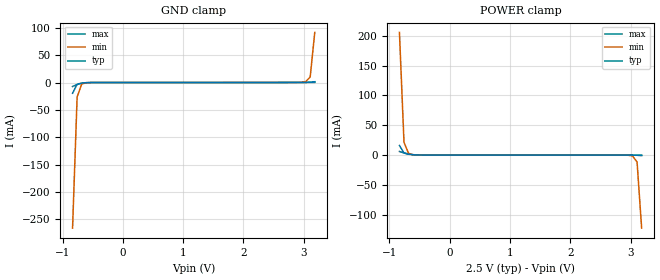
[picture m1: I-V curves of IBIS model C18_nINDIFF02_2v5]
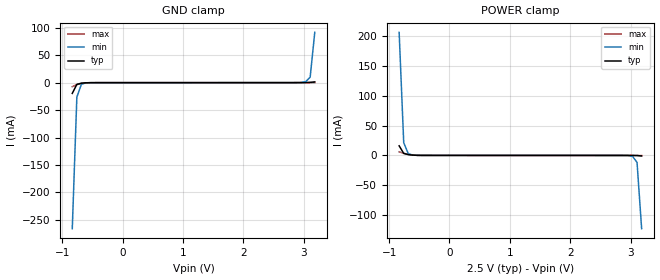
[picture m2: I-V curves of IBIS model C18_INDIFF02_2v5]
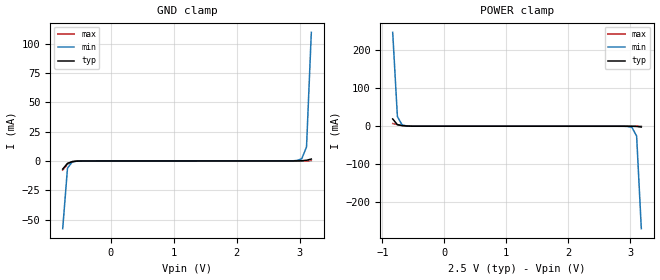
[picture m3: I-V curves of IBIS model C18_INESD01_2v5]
|   This file is an IBIS representation of the   |
|   Integrated Device Technology, Inc.   |
|   8L30210I   |
|   CRYSTAL OR DIFFERENTIAL-TO-LVCMOS LVTTL CLOCK BUFFER   |
[IBIS Ver]   4.1
[File name]   8l30210i.ibs
[File Rev]   1.0
[Date]   04 Dec 2019
[Source]   Originated at Integrated Device Technology, Inc.
[Disclaimer]
IDT hereby grants the user of this IBIS model a non-exclusive,
nontransferable license to use this IBIS model under the following terms.
Before using this IBIS model, the user should read this license.
If the user does not accept these terms,  the IBIS model should be
returned to IDT within 30 days.
   The user is granted this license only to use the IBIS model and
is not granted rights to sell, load, rent, lease or license the IBIS
model in whole or in part, or in modified form to anyone other than
user. User may modify the IBIS model to suit its specific
applications but rights to derivative works and such modifications
shall belong to IDT.
   This IBIS model is provided on an "AS IS" basis and IDT makes
absolutely no warranty with respect to the information contained
herein. IDT DISCLAIMS AND CUSTOMER WAIVES ALL WARRANTIES, EXPRESS
OR IMPLIED, INCLUDING WARRANTIES OF MERCHANTABILITY OR FITNESS FOR
A PARTICULAR PURPOSE. The entire risk as to quality and performance
is with the Customer. ACCORDINGLY, IN NO EVENT SHALL THE COMPANY BE
LIABLE FOR ANY DAMAGES, WHETHER IN CONTRACT OR TORT,INCLUDING ANY
LOST PROFITS OR OTHER INCIDENTAL, CONSEQUENTIAL, EXEMPLARY, OR
PUNITIVE DAMAGES ARISING OUT OF THE USE OR APPLICATION OF THE IBIS
model provided in this package. Further, IDT reserves the right to
make changes without notice to any product herein to improve
reliability, function, or design. IDT does not convey any license
under patent rights or any other intellectual property rights,
including those of third parties.
   IDT is not obligated to provide maintenance or support
for the licensed IBIS model.
[Copyright] Copyright 2019 by Integrated Device Technology, Inc.
[Component]   8L30210NLGI
[Manufacturer] Integrated Device Technology, Inc.
[Package]
|QFN 32
|lead + wire   typ   min   max
R_pkg   72.4655m   58.886m   86.045m
L_pkg   1.47175nH   1.11650nH   1.77850nH
C_pkg   0.07747pF   0.07444pF   0.08050pF
[Pin] signal_name   model_name   R_pin   L_pin   C_pin
1   Q0   c18_OCMOS50OHM09   86.045m   1.77850nH   0.08050pF
2   VDDO   POWER   76.996m   1.55783nH   0.07848pF
3   Q1   c18_OCMOS50OHM09   67.941m   1.33717nH   0.07646pF
4   GND0   GND   58.886m   1.11650nH   0.07444pF
5   Q2   c18_OCMOS50OHM09   58.886m   1.11650nH   0.07444pF
6   VDDO   POWER   67.941m   1.33717nH   0.07646pF
7   Q3   c18_OCMOS50OHM09   76.996m   1.55783nH   0.07848pF
8   Q4   c18_OCMOS50OHM09   86.045m   1.77850nH   0.08050pF
9   GND0   GND   86.045m   1.77850nH   0.08050pF
10   VDD   POWER   76.996m   1.55783nH   0.07848pF
11   XTAL_IN   NC   67.941m   1.33717nH   0.07646pF
12   XTAL_OUT   NC   58.886m   1.11650nH   0.07444pF
13   CLK0   C18_INDIFF02   58.886m   1.11650nH   0.07444pF
14   nCLK0   C18_nINDIFF02   67.941m   1.33717nH   0.07646pF
15   GND   GND   76.996m   1.55783nH   0.07848pF
16   GND0   GND   86.045m   1.77850nH   0.08050pF
17   Q5   c18_OCMOS50OHM09   86.045m   1.77850nH   0.08050pF
18   Q6   c18_OCMOS50OHM09   76.996m   1.55783nH   0.07848pF
19   VDD0   POWER   67.941m   1.33717nH   0.07646pF
20   Q7   c18_OCMOS50OHM09   58.886m   1.11650nH   0.07444pF
21   GND0   GND   58.886m   1.11650nH   0.07444pF
22   Q8   c18_OCMOS50OHM09   67.941m   1.33717nH   0.07646pF
23   VDDO   POWER   76.996m   1.55783nH   0.07848pF
24   Q9   c18_OCMOS50OHM09   86.045m   1.77850nH   0.08050pF
25   GND0   GND   86.045m   1.77850nH   0.08050pF
26   GND   GND   76.996m   1.55783nH   0.07848pF
27   nCLK1   C18_nINDIFF02   67.941m   1.33717nH   0.07646pF
28   CLK1   C18_INDIFF02   58.886m   1.11650nH   0.07444pF
29   SEL1   C18_INESD01   58.886m   1.11650nH   0.07444pF
30   SEL0   C18_INESD01   67.941m   1.33717nH   0.07646pF
31   OE   C18_INESD01   76.996m   1.55783nH   0.07848pF
32   GND0   GND   86.045m   1.77850nH   0.08050pF
[Diff Pin]  inv_pin  vdiff tdelay_typ tdelay_min  tdelay_max
13   14   0.15   NA   NA   NA
28   27   0.15   NA   NA   NA
[Model Selector] c18_OCMOS50OHM09
c18_OCMOS50OHM09_1v5  Buffer selection for 1v5
c18_OCMOS50OHM09_1v8  Buffer selection for 1v8
c18_OCMOS50OHM09_2v5  Buffer selection for 2v5
c18_OCMOS50OHM09_3v3  Buffer selection for 3v3
[Model Selector] C18_nINDIFF02
C18_nINDIFF02_2v5  Buffer selection for 2v5
C18_nINDIFF02_3v3  Buffer selection for 3v3
[Model Selector] C18_INDIFF02
C18_INDIFF02_2v5  Buffer selection for 2v5
C18_INDIFF02_3v3  Buffer selection for 3v3
[Model Selector] C18_INESD01
C18_INESD01_2v5  Buffer selection for 2v5
C18_INESD01_3v3  Buffer selection for 3v3
| Models and submodels in the file (10): C18_nINDIFF02_2v5 (Input), C18_INDIFF02_2v5 (Input), C18_INESD01_2v5 (Input), c18_OCMOS50OHM09_1v5 (Output), c18_OCMOS50OHM09_1v8 (Output), c18_OCMOS50OHM09_2v5 (Output), c18_OCMOS50OHM09_3v3 (Output), C18_nINDIFF02_3v3 (Input), C18_INDIFF02_3v3 (Input), C18_INESD01_3v3 (Input)
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[Model] C18_nINDIFF02_2v5
Model_type   Input
Polarity   Non-Inverting
Vinl = 0.7V
Vinh = 1.7V
|   typ   min   max
C_comp   2pF   1.5pF   2.5pF
|   typ   min   max
[Voltage range]   2.5V   2.375V   2.625V
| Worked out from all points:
|   GND clamp passes 1 mA (typ) near -0.68 V on its own axis
|   POWER clamp passes 1 mA (typ) near -0.65 V on its own axis
[GND_clamp]
|Voltage   I (typ)   I (min)   I (max)
|Note, modeling breaks down at 250mA and above.  This is well beyond the functional   |
|operating range of the device.  Should this scenario occur, catastrophic failure and   |
|possible damage to the device and/or board is of higher concern than the I-V curve   |
|behavior.  The IBIS checker will flag currents in excess of 10A with warnings.  Lines   |
|with currents in excess of 0.35 A have been commented out.  The points still remain|
|available to the user if the user desires to use them.   |
|-2.50000e+00   -1.17752e+01   -1.02957e+01   -1.42772e+01
|-2.42424e+00   -1.12274e+01   -9.83984e+00   -1.35771e+01
|-2.34848e+00   -1.06796e+01   -9.38392e+00   -1.28769e+01
|-2.27273e+00   -1.01318e+01   -8.92797e+00   -1.21767e+01
|-2.19697e+00   -9.58387e+00   -8.47198e+00   -1.14763e+01
|-2.12121e+00   -9.03588e+00   -8.01595e+00   -1.07758e+01
|-2.04545e+00   -8.48784e+00   -7.55989e+00   -1.00752e+01
|-1.96970e+00   -7.93974e+00   -7.10380e+00   -9.37454e+00
|-1.89394e+00   -7.39159e+00   -6.64768e+00   -8.67378e+00
|-1.81818e+00   -6.84339e+00   -6.19154e+00   -7.97293e+00
|-1.74242e+00   -6.29514e+00   -5.73539e+00   -7.27199e+00
|-1.66667e+00   -5.74687e+00   -5.27924e+00   -6.57098e+00
|-1.59091e+00   -5.19857e+00   -4.82308e+00   -5.86989e+00
|-1.51515e+00   -4.65027e+00   -4.36695e+00   -5.16875e+00
|-1.43939e+00   -4.10197e+00   -3.91083e+00   -4.46756e+00
|-1.36364e+00   -3.55369e+00   -3.45477e+00   -3.76634e+00
|-1.28788e+00   -3.00546e+00   -2.99876e+00   -3.06512e+00
|-1.21212e+00   -2.45731e+00   -2.54285e+00   -2.36393e+00
|-1.13636e+00   -1.90928e+00   -2.08704e+00   -1.66282e+00
|-1.06061e+00   -1.36142e+00   -1.63139e+00   -9.61838e-01
|-9.84848e-01   -8.13796e-01   -1.17595e+00   -2.61081e-01
|-9.09091e-01   -2.66503e-01   -7.20781e-01   -1.77649e-02
-833.3mV  -19.6mA    -266mA     -7.357mA
-757.6mV  -3.22mA    -26.35mA   -3.621mA
-681.8mV  -988.6uA   -2.843mA   -1.31mA
-530.3mV  -114.3uA   -121.3uA   -118.4uA
2.803V    62.2uA     69.71uA    63.29uA
3.03V     168.3uA    1.59mA     74.62uA
3.106V    527.5uA    10.07mA    99.45uA
3.182V    1.407mA    91.57mA    275.1uA
| 3.25758e+00   3.38287e-03   7.21084e-01   9.53838e-04
| 3.33333e+00   1.60717e-02   1.60186e+00   2.32699e-03
| 3.40909e+00   2.04604e-01   2.48284e+00   4.31441e-03
| 3.48485e+00   1.20201e+00   3.36401e+00   7.22826e-03
| 3.56061e+00   2.26050e+00   4.24535e+00   2.70580e-02
| 3.63636e+00   3.31920e+00   5.12684e+00   5.94903e-01
| 3.71212e+00   4.37810e+00   6.00848e+00   1.94867e+00
| 3.78788e+00   5.43717e+00   6.89026e+00   3.30270e+00
| 3.86364e+00   6.49642e+00   7.77218e+00   4.65695e+00
| 3.93939e+00   7.55581e+00   8.65422e+00   6.01139e+00
| 4.01515e+00   8.61535e+00   9.53640e+00   7.36602e+00
| 4.09091e+00   9.67503e+00   1.04187e+01   8.72081e+00
| 4.16667e+00   1.07348e+01   1.13011e+01   1.00758e+01
| 4.24242e+00   1.17948e+01   1.21837e+01   1.14308e+01
| 4.31818e+00   1.28549e+01   1.30664e+01   1.27860e+01
| 4.39394e+00   1.39151e+01   1.39493e+01   1.41414e+01
| 4.46970e+00   1.49754e+01   1.48323e+01   1.54969e+01
| 4.54545e+00   1.60359e+01   1.57155e+01   1.68525e+01
| 4.62121e+00   1.70966e+01   1.65988e+01   1.82082e+01
| 4.69697e+00   1.81574e+01   1.74824e+01   1.95641e+01
| 4.77273e+00   1.92184e+01   1.83662e+01   2.09201e+01
| 4.84848e+00   2.02796e+01   1.92502e+01   2.22763e+01
| 4.92424e+00   2.13410e+01   2.01345e+01   2.36327e+01
| 5.00000e+00   2.24026e+01   2.10190e+01   2.49892e+01
[Power_clamp]
|Voltage   I (typ)   I (min)   I (max)
|Note, modeling breaks down at 250mA and above.  This is well beyond the functional   |
|operating range of the device.  Should this scenario occur, catastrophic failure and   |
|possible damage to the device and/or board is of higher concern than the I-V curve   |
|behavior.  The IBIS checker will flag currents in excess of 10A with warnings.  Lines   |
|with currents in excess of 0.35 A have been commented out.  The points still remain|
|available to the user if the user desires to use them.   |
|-2.50000e+00   2.24026e+01   1.95597e+01   2.72279e+01
|-2.42424e+00   2.13410e+01   1.86756e+01   2.58711e+01
|-2.34848e+00   2.02796e+01   1.77917e+01   2.45144e+01
|-2.27273e+00   1.92184e+01   1.69081e+01   2.31579e+01
|-2.19697e+00   1.81574e+01   1.60246e+01   2.18016e+01
|-2.12121e+00   1.70966e+01   1.51414e+01   2.04455e+01
|-2.04545e+00   1.60359e+01   1.42583e+01   1.90895e+01
|-1.96970e+00   1.49754e+01   1.33754e+01   1.77337e+01
|-1.89394e+00   1.39151e+01   1.24926e+01   1.63780e+01
|-1.81818e+00   1.28549e+01   1.16100e+01   1.50224e+01
|-1.74242e+00   1.17948e+01   1.07275e+01   1.36670e+01
|-1.66667e+00   1.07348e+01   9.84519e+00   1.23117e+01
|-1.59091e+00   9.67503e+00   8.96297e+00   1.09565e+01
|-1.51515e+00   8.61535e+00   8.08088e+00   9.60151e+00
|-1.43939e+00   7.55581e+00   7.19892e+00   8.24662e+00
|-1.36364e+00   6.49642e+00   6.31709e+00   6.89188e+00
|-1.28788e+00   5.43717e+00   5.43540e+00   5.53732e+00
|-1.21212e+00   4.37810e+00   4.55385e+00   4.18293e+00
|-1.13636e+00   3.31920e+00   3.67246e+00   2.82876e+00
|-1.06061e+00   2.26050e+00   2.79123e+00   1.47482e+00
|-9.84848e-01   1.20201e+00   1.91018e+00   1.95536e-01
|-9.09091e-01   2.04604e-01   1.02933e+00   1.34857e-02
-833.3mV  16.07mA    205.9mA    5.983mA
-757.6mV  3.383mA    21.22mA    3.554mA
-681.8mV  1.407mA    2.877mA    1.771mA
-606.1mV  527.5uA    600.2uA    638.2uA
-454.5mV  81.85uA    79.3uA     84.87uA
2.879V    -65.87uA   -93.69uA   -66.51uA
3.03V     -114.3uA   -1.397mA   -73.64uA
3.106V    -301.2uA   -11.78mA   -85.59uA
3.182V    -988.6uA   -122.6mA   -160.7uA
| 3.25758e+00   -3.21985e-03   -5.61557e-01   -5.63528e-04
| 3.33333e+00   -1.95987e-02   -1.01660e+00   -1.95169e-03
| 3.40909e+00   -2.66503e-01   -1.47196e+00   -4.76211e-03
| 3.48485e+00   -8.13796e-01   -1.92755e+00   -9.23293e-03
| 3.56061e+00   -1.36142e+00   -2.38330e+00   -3.58634e-02
| 3.63636e+00   -1.90928e+00   -2.83918e+00   -5.06314e-01
| 3.71212e+00   -2.45731e+00   -3.29516e+00   -1.20716e+00
| 3.78788e+00   -3.00546e+00   -3.75121e+00   -1.90820e+00
| 3.86364e+00   -3.55369e+00   -4.20730e+00   -2.60934e+00
| 3.93939e+00   -4.10197e+00   -4.66343e+00   -3.31055e+00
| 4.01515e+00   -4.65027e+00   -5.11958e+00   -4.01177e+00
| 4.09091e+00   -5.19857e+00   -5.57574e+00   -4.71298e+00
| 4.16667e+00   -5.74687e+00   -6.03189e+00   -5.41416e+00
| 4.24242e+00   -6.29514e+00   -6.48804e+00   -6.11528e+00
| 4.31818e+00   -6.84339e+00   -6.94416e+00   -6.81634e+00
| 4.39394e+00   -7.39159e+00   -7.40026e+00   -7.51733e+00
| 4.46970e+00   -7.93974e+00   -7.85633e+00   -8.21823e+00
| 4.54545e+00   -8.48784e+00   -8.31238e+00   -8.91906e+00
| 4.62121e+00   -9.03588e+00   -8.76838e+00   -9.61979e+00
| 4.69697e+00   -9.58387e+00   -9.22435e+00   -1.03204e+01
| 4.77273e+00   -1.01318e+01   -9.68027e+00   -1.10210e+01
| 4.84848e+00   -1.06796e+01   -1.01362e+01   -1.17214e+01
| 4.92424e+00   -1.12274e+01   -1.05920e+01   -1.24218e+01
| 5.00000e+00   -1.17752e+01   -1.10478e+01   -1.31220e+01
[Model] C18_INDIFF02_2v5
Model_type   Input
Polarity   Non-Inverting
Vinl = 0.7V
Vinh = 1.7V
|   typ   min   max
C_comp   2pF   1.5pF   2.5pF
|   typ   min   max
[Voltage range]   2.5V   2.375V   2.625V
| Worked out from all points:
|   GND clamp passes 1 mA (typ) near -0.68 V on its own axis
|   POWER clamp passes 1 mA (typ) near -0.65 V on its own axis
[GND_clamp]
|Voltage   I (typ)   I (min)   I (max)
|Note, modeling breaks down at 250mA and above.  This is well beyond the functional   |
|operating range of the device.  Should this scenario occur, catastrophic failure and   |
|possible damage to the device and/or board is of higher concern than the I-V curve   |
|behavior.  The IBIS checker will flag currents in excess of 10A with warnings.  Lines   |
|with currents in excess of 0.35 A have been commented out.  The points still remain|
|available to the user if the user desires to use them.   |
|-2.50000e+00   -1.17751e+01   -1.02956e+01   -1.42771e+01
|-2.42424e+00   -1.12273e+01   -9.83975e+00   -1.35770e+01
|-2.34848e+00   -1.06795e+01   -9.38384e+00   -1.28768e+01
|-2.27273e+00   -1.01317e+01   -8.92789e+00   -1.21765e+01
|-2.19697e+00   -9.58377e+00   -8.47190e+00   -1.14762e+01
|-2.12121e+00   -9.03579e+00   -8.01587e+00   -1.07757e+01
|-2.04545e+00   -8.48775e+00   -7.55981e+00   -1.00751e+01
|-1.96970e+00   -7.93965e+00   -7.10372e+00   -9.37444e+00
|-1.89394e+00   -7.39150e+00   -6.64760e+00   -8.67368e+00
|-1.81818e+00   -6.84330e+00   -6.19147e+00   -7.97283e+00
|-1.74242e+00   -6.29506e+00   -5.73532e+00   -7.27190e+00
|-1.66667e+00   -5.74679e+00   -5.27916e+00   -6.57089e+00
|-1.59091e+00   -5.19849e+00   -4.82301e+00   -5.86980e+00
|-1.51515e+00   -4.65019e+00   -4.36687e+00   -5.16866e+00
|-1.43939e+00   -4.10189e+00   -3.91076e+00   -4.46747e+00
|-1.36364e+00   -3.55361e+00   -3.45470e+00   -3.76626e+00
|-1.28788e+00   -3.00539e+00   -2.99869e+00   -3.06504e+00
|-1.21212e+00   -2.45724e+00   -2.54278e+00   -2.36385e+00
|-1.13636e+00   -1.90921e+00   -2.08698e+00   -1.66274e+00
|-1.06061e+00   -1.36135e+00   -1.63133e+00   -9.61760e-01
|-9.84848e-01   -8.13726e-01   -1.17589e+00   -2.61004e-01
|-9.09091e-01   -2.66435e-01   -7.20720e-01   -1.76899e-02
-833.3mV  -19.53mA   -265.9mA   -7.283mA
-757.6mV  -3.155mA   -26.29mA   -3.549mA
-681.8mV  -925uA     -2.786mA   -1.24mA
-530.3mV  -53.72uA   -66.97uA   -51.38uA
2.803V    56.14uA    61.7uA     59.51uA
3.03V     157.7uA    1.578mA    66.02uA
3.106V    515.4uA    10.06mA    89.24uA
3.182V    1.393mA    91.56mA    263.3uA
| 3.25758e+00   3.36773e-03   7.21068e-01   9.40408e-04
| 3.33333e+00   1.60551e-02   1.60184e+00   2.31196e-03
| 3.40909e+00   2.04586e-01   2.48282e+00   4.29776e-03
| 3.48485e+00   1.20199e+00   3.36399e+00   7.21000e-03
| 3.56061e+00   2.26047e+00   4.24533e+00   2.70381e-02
| 3.63636e+00   3.31917e+00   5.12682e+00   5.94881e-01
| 3.71212e+00   4.37807e+00   6.00846e+00   1.94865e+00
| 3.78788e+00   5.43715e+00   6.89024e+00   3.30267e+00
| 3.86364e+00   6.49639e+00   7.77215e+00   4.65692e+00
| 3.93939e+00   7.55578e+00   8.65419e+00   6.01137e+00
| 4.01515e+00   8.61532e+00   9.53637e+00   7.36599e+00
| 4.09091e+00   9.67500e+00   1.04187e+01   8.72078e+00
| 4.16667e+00   1.07348e+01   1.13011e+01   1.00757e+01
| 4.24242e+00   1.17948e+01   1.21837e+01   1.14308e+01
| 4.31818e+00   1.28548e+01   1.30664e+01   1.27860e+01
| 4.39394e+00   1.39150e+01   1.39492e+01   1.41414e+01
| 4.46970e+00   1.49754e+01   1.48323e+01   1.54968e+01
| 4.54545e+00   1.60359e+01   1.57154e+01   1.68524e+01
| 4.62121e+00   1.70965e+01   1.65988e+01   1.82082e+01
| 4.69697e+00   1.81574e+01   1.74824e+01   1.95641e+01
| 4.77273e+00   1.92184e+01   1.83661e+01   2.09201e+01
| 4.84848e+00   2.02795e+01   1.92502e+01   2.22763e+01
| 4.92424e+00   2.13409e+01   2.01344e+01   2.36326e+01
| 5.00000e+00   2.24025e+01   2.10190e+01   2.49892e+01
[Power_clamp]
|Voltage   I (typ)   I (min)   I (max)
|Note, modeling breaks down at 250mA and above.  This is well beyond the functional   |
|operating range of the device.  Should this scenario occur, catastrophic failure and   |
|possible damage to the device and/or board is of higher concern than the I-V curve   |
|behavior.  The IBIS checker will flag currents in excess of 10A with warnings.  Lines   |
|with currents in excess of 0.35 A have been commented out.  The points still remain|
|available to the user if the user desires to use them.   |
|-2.50000e+00   2.24025e+01   1.95596e+01   2.72279e+01
|-2.42424e+00   2.13409e+01   1.86755e+01   2.58710e+01
|-2.34848e+00   2.02795e+01   1.77917e+01   2.45144e+01
|-2.27273e+00   1.92184e+01   1.69080e+01   2.31579e+01
|-2.19697e+00   1.81574e+01   1.60246e+01   2.18016e+01
|-2.12121e+00   1.70965e+01   1.51413e+01   2.04455e+01
|-2.04545e+00   1.60359e+01   1.42583e+01   1.90895e+01
|-1.96970e+00   1.49754e+01   1.33754e+01   1.77337e+01
|-1.89394e+00   1.39150e+01   1.24926e+01   1.63780e+01
|-1.81818e+00   1.28548e+01   1.16100e+01   1.50224e+01
|-1.74242e+00   1.17948e+01   1.07275e+01   1.36670e+01
|-1.66667e+00   1.07348e+01   9.84516e+00   1.23117e+01
|-1.59091e+00   9.67500e+00   8.96294e+00   1.09565e+01
|-1.51515e+00   8.61532e+00   8.08085e+00   9.60148e+00
|-1.43939e+00   7.55578e+00   7.19889e+00   8.24659e+00
|-1.36364e+00   6.49639e+00   6.31706e+00   6.89185e+00
|-1.28788e+00   5.43715e+00   5.43537e+00   5.53729e+00
|-1.21212e+00   4.37807e+00   4.55383e+00   4.18291e+00
|-1.13636e+00   3.31917e+00   3.67244e+00   2.82874e+00
|-1.06061e+00   2.26047e+00   2.79121e+00   1.47480e+00
|-9.84848e-01   1.20199e+00   1.91016e+00   1.95515e-01
|-9.09091e-01   2.04586e-01   1.02931e+00   1.34664e-02
-833.3mV  16.06mA    205.8mA    5.965mA
-757.6mV  3.368mA    21.21mA    3.538mA
-681.8mV  1.393mA    2.864mA    1.756mA
-606.1mV  515.4uA    588.8uA    625.4uA
-454.5mV  72.76uA    70.8uA     75.22uA
2.879V    -8.33uA    -39.85uA   -5.39uA
3.03V     -53.72uA   -1.341mA   -9.307uA
3.106V    -239.1uA   -11.72mA   -19.64uA
3.182V    -925uA     -122.5mA   -93.12uA
| 3.25758e+00   -3.15473e-03   -5.61496e-01   -4.94368e-04
| 3.33333e+00   -1.95321e-02   -1.01654e+00   -1.88092e-03
| 3.40909e+00   -2.66435e-01   -1.47190e+00   -4.68973e-03
| 3.48485e+00   -8.13726e-01   -1.92748e+00   -9.15894e-03
| 3.56061e+00   -1.36135e+00   -2.38323e+00   -3.57878e-02
| 3.63636e+00   -1.90921e+00   -2.83911e+00   -5.06236e-01
| 3.71212e+00   -2.45724e+00   -3.29509e+00   -1.20708e+00
| 3.78788e+00   -3.00539e+00   -3.75113e+00   -1.90812e+00
| 3.86364e+00   -3.55361e+00   -4.20723e+00   -2.60926e+00
| 3.93939e+00   -4.10189e+00   -4.66336e+00   -3.31047e+00
| 4.01515e+00   -4.65019e+00   -5.11951e+00   -4.01169e+00
| 4.09091e+00   -5.19849e+00   -5.57566e+00   -4.71289e+00
| 4.16667e+00   -5.74679e+00   -6.03181e+00   -5.41407e+00
| 4.24242e+00   -6.29506e+00   -6.48796e+00   -6.11519e+00
| 4.31818e+00   -6.84330e+00   -6.94408e+00   -6.81625e+00
| 4.39394e+00   -7.39150e+00   -7.40018e+00   -7.51723e+00
| 4.46970e+00   -7.93965e+00   -7.85625e+00   -8.21814e+00
| 4.54545e+00   -8.48775e+00   -8.31229e+00   -8.91896e+00
| 4.62121e+00   -9.03579e+00   -8.76829e+00   -9.61969e+00
| 4.69697e+00   -9.58377e+00   -9.22426e+00   -1.03203e+01
| 4.77273e+00   -1.01317e+01   -9.68018e+00   -1.10209e+01
| 4.84848e+00   -1.06795e+01   -1.01361e+01   -1.17213e+01
| 4.92424e+00   -1.12273e+01   -1.05919e+01   -1.24217e+01
| 5.00000e+00   -1.17751e+01   -1.10477e+01   -1.31219e+01
[Model] C18_INESD01_2v5
Model_type   Input
Polarity   Non-Inverting
Vinl = 0.7V
Vinh = 1.7V
|   typ   min   max
C_comp   2pF   1.5pF   2.5pF
|   typ   min   max
[Voltage range]   2.5V   2.375V   2.625V
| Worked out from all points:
|   GND clamp passes 1 mA (typ) near -0.63 V on its own axis
|   POWER clamp passes 1 mA (typ) near -0.63 V on its own axis
[GND_clamp]
|Voltage   I (typ)   I (min)   I (max)
|Note, modeling breaks down at 250mA and above.  This is well beyond the functional   |
|operating range of the device.  Should this scenario occur, catastrophic failure and   |
|possible damage to the device and/or board is of higher concern than the I-V curve   |
|behavior.  The IBIS checker will flag currents in excess of 10A with warnings.  Lines   |
|with currents in excess of 0.35 A have been commented out.  The points still remain|
|available to the user if the user desires to use them.   |
|-2.50000e+00   -2.59051e+01   -2.26503e+01   -3.14096e+01
|-2.42424e+00   -2.47001e+01   -2.16474e+01   -2.98694e+01
|-2.34848e+00   -2.34950e+01   -2.06444e+01   -2.83290e+01
|-2.27273e+00   -2.22897e+01   -1.96413e+01   -2.67883e+01
|-2.19697e+00   -2.10843e+01   -1.86381e+01   -2.52475e+01
|-2.12121e+00   -1.98787e+01   -1.76349e+01   -2.37065e+01
|-2.04545e+00   -1.86730e+01   -1.66315e+01   -2.21652e+01
|-1.96970e+00   -1.74672e+01   -1.56281e+01   -2.06237e+01
|-1.89394e+00   -1.62613e+01   -1.46247e+01   -1.90821e+01
|-1.81818e+00   -1.50552e+01   -1.36212e+01   -1.75402e+01
|-1.74242e+00   -1.38491e+01   -1.26177e+01   -1.59981e+01
|-1.66667e+00   -1.26429e+01   -1.16141e+01   -1.44559e+01
|-1.59091e+00   -1.14366e+01   -1.06106e+01   -1.29135e+01
|-1.51515e+00   -1.02304e+01   -9.60709e+00   -1.13710e+01
|-1.43939e+00   -9.02412e+00   -8.60365e+00   -9.82840e+00
|-1.36364e+00   -7.81792e+00   -7.60030e+00   -8.28573e+00
|-1.28788e+00   -6.61182e+00   -6.59710e+00   -6.74306e+00
|-1.21212e+00   -5.40590e+00   -5.59409e+00   -5.20044e+00
|-1.13636e+00   -4.20024e+00   -4.59132e+00   -3.65800e+00
|-1.06061e+00   -2.99495e+00   -3.58890e+00   -2.11585e+00
|-9.84848e-01   -1.79017e+00   -2.58693e+00   -5.74184e-01
|-9.09091e-01   -5.86135e-01   -1.58556e+00   -3.88946e-02
|-8.33333e-01   -4.29506e-02   -5.85049e-01   -1.60019e-02
-757.6mV  -6.922mA   -57.82mA   -7.788mA
-681.8mV  -2.019mA   -6.114mA   -2.71mA
-606.1mV  -511.5uA   -812.7uA   -604.9uA
-454.5mV  -23.28uA   -29.32uA   -18.42uA
2.803V    56.17uA    63.56uA    59.51uA
2.955V    75.5uA     423.2uA    62.82uA
3.03V     177.1uA    1.883mA    66.35uA
3.106V    606uA      12.06mA    93.9uA
3.182V    1.659mA    109.9mA    302.4uA
| 3.25758e+00   4.02825e-03   8.65269e-01   1.11466e-03
| 3.33333e+00   1.92528e-02   1.92220e+00   2.76019e-03
| 3.40909e+00   2.45489e-01   2.97938e+00   5.14284e-03
| 3.48485e+00   1.44238e+00   4.03678e+00   8.63721e-03
| 3.56061e+00   2.71256e+00   5.09438e+00   3.24306e-02
| 3.63636e+00   3.98300e+00   6.15217e+00   7.13842e-01
| 3.71212e+00   5.25367e+00   7.21013e+00   2.33836e+00
| 3.78788e+00   6.52456e+00   8.26827e+00   3.96319e+00
| 3.86364e+00   7.79565e+00   9.32656e+00   5.58829e+00
| 3.93939e+00   9.06692e+00   1.03850e+01   7.21362e+00
| 4.01515e+00   1.03384e+01   1.14436e+01   8.83917e+00
| 4.09091e+00   1.16100e+01   1.25024e+01   1.04649e+01
| 4.16667e+00   1.28818e+01   1.35613e+01   1.20908e+01
| 4.24242e+00   1.41537e+01   1.46204e+01   1.37169e+01
| 4.31818e+00   1.54258e+01   1.56796e+01   1.53432e+01
| 4.39394e+00   1.66980e+01   1.67391e+01   1.69696e+01
| 4.46970e+00   1.79705e+01   1.77987e+01   1.85962e+01
| 4.54545e+00   1.92431e+01   1.88585e+01   2.02229e+01
| 4.62121e+00   2.05158e+01   1.99185e+01   2.18498e+01
| 4.69697e+00   2.17888e+01   2.09788e+01   2.34769e+01
| 4.77273e+00   2.30620e+01   2.20393e+01   2.51041e+01
| 4.84848e+00   2.43354e+01   2.31002e+01   2.67315e+01
| 4.92424e+00   2.56091e+01   2.41613e+01   2.83591e+01
| 5.00000e+00   2.68830e+01   2.52228e+01   2.99870e+01
[Power_clamp]
|Voltage   I (typ)   I (min)   I (max)
|Note, modeling breaks down at 250mA and above.  This is well beyond the functional   |
|operating range of the device.  Should this scenario occur, catastrophic failure and   |
|possible damage to the device and/or board is of higher concern than the I-V curve   |
|behavior.  The IBIS checker will flag currents in excess of 10A with warnings.  Lines   |
|with currents in excess of 0.35 A have been commented out.  The points still remain|
|available to the user if the user desires to use them.   |
|-2.50000e+00   2.68830e+01   2.34715e+01   3.26734e+01
|-2.42424e+00   2.56091e+01   2.24106e+01   3.10452e+01
|-2.34848e+00   2.43354e+01   2.13500e+01   2.94172e+01
|-2.27273e+00   2.30620e+01   2.02896e+01   2.77894e+01
|-2.19697e+00   2.17888e+01   1.92295e+01   2.61619e+01
|-2.12121e+00   2.05158e+01   1.81696e+01   2.45345e+01
|-2.04545e+00   1.92431e+01   1.71099e+01   2.29074e+01
|-1.96970e+00   1.79705e+01   1.60504e+01   2.12804e+01
|-1.89394e+00   1.66980e+01   1.49911e+01   1.96535e+01
|-1.81818e+00   1.54258e+01   1.39320e+01   1.80269e+01
|-1.74242e+00   1.41537e+01   1.28730e+01   1.64003e+01
|-1.66667e+00   1.28818e+01   1.18142e+01   1.47740e+01
|-1.59091e+00   1.16100e+01   1.07555e+01   1.31478e+01
|-1.51515e+00   1.03384e+01   9.69701e+00   1.15218e+01
|-1.43939e+00   9.06692e+00   8.63865e+00   9.89589e+00
|-1.36364e+00   7.79565e+00   7.58046e+00   8.27021e+00
|-1.28788e+00   6.52456e+00   6.52244e+00   6.64473e+00
|-1.21212e+00   5.25367e+00   5.46458e+00   5.01947e+00
|-1.13636e+00   3.98300e+00   4.40691e+00   3.39447e+00
|-1.06061e+00   2.71256e+00   3.34944e+00   1.76974e+00
|-9.84848e-01   1.44238e+00   2.29219e+00   2.34603e-01
|-9.09091e-01   2.45489e-01   1.23516e+00   1.61447e-02
-833.3mV  19.25mA    247mA      7.144mA
-757.6mV  4.028mA    25.44mA    4.231mA
-681.8mV  1.659mA    3.425mA    2.094mA
-530.3mV  177.1uA    181uA      185.8uA
2.879V    -9.239uA   -76.38uA   -5.392uA
3.03V     -105.5uA   -2.935mA   -10.15uA
3.106V    -511.5uA   -25.77mA   -30.96uA
3.182V    -2.019mA   -269.5mA   -190.7uA
